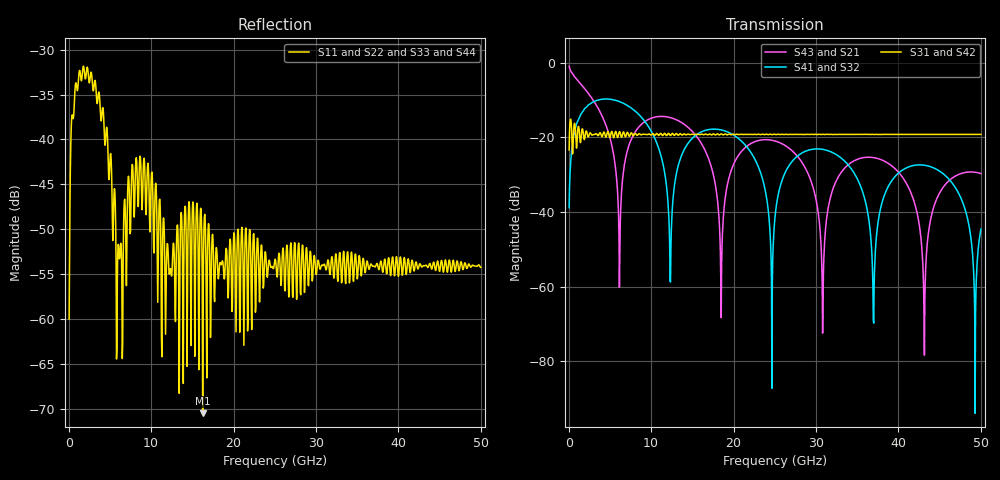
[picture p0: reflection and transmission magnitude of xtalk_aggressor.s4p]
! Created with skrf 1.10.0 (http://scikit-rf.org).
# GHz S RI R 50.0
!freq ReS11 ImS11 ReS12 ImS12 ReS13 ImS13
! ReS14 ImS14
! ReS21 ImS21 ReS22 ImS22 ReS23 ImS23
! ReS24 ImS24
! ReS31 ImS31 ReS32 ImS32 ReS33 ImS33
! ReS34 ImS34
! ReS41 ImS41 ReS42 ImS42 ReS43 ImS43
! ReS44 ImS44
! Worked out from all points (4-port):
!   1000 points, 50 MHz to 50 GHz, reference 50 ohm
!   strongest paths, dB at 50 MHz, 12.55 GHz, 25.05 GHz, 37.55 GHz, 50 GHz:
!     S31: -23.4, -19.0, -19.2, -19.3, -19.2
!     S42: -23.4, -19.0, -19.2, -19.3, -19.2
!     S41: -38.9, -39.7, -40.8, -42.4, -44.6
!     S32: -38.9, -39.7, -40.8, -42.4, -44.6
!     S43: -1.0, -14.9, -21.0, -25.7, -29.7
!     S21: -1.0, -14.9, -21.0, -25.7, -29.7
!   lowest |S11| = -70.4 dB at 16.25 GHz (marker M1), VSWR 1.00, Z = 50 + j0.0298 ohm
!   |S11| at or under -10 dB: start of sweep to end of sweep
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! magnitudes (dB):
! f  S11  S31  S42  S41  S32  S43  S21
! 50 MHz  -60.0  -23.4  -23.4  -38.9  -38.9  -1.0  -1.0
! 6.15 GHz  -53.3  -18.5  -18.5  -10.5  -10.5  -60.1  -60.1
! 12.3 GHz  -54.4  -19.5  -19.5  -58.5  -58.5  -14.7  -14.7
! 16.25 GHz  -70.4  -19.2  -19.2  -18.4  -18.4  -22.3  -22.3
! 24.65 GHz  -54.1  -19.3  -19.3  -87.2  -87.2  -20.8  -20.8
! 43.15 GHz  -54.0  -19.2  -19.2  -27.5  -27.5  -78.3  -78.3
! 50 GHz  -54.2  -19.2  -19.2  -44.6  -44.6  -29.7  -29.7
